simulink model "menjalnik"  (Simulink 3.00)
settings: Solver=ode45  StartTime=0.0  StopTime=100.0  RelTol=1e-3

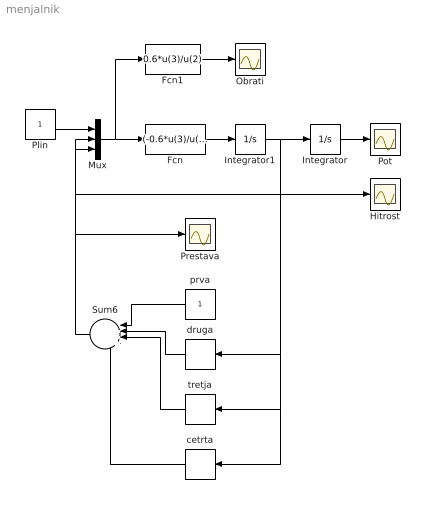
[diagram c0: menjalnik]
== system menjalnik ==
  Fcn : Fcn  Expr=(-0.6*u(3)/u(2)+u(1))/(1+u(2))
  Fcn1 : Fcn  Expr=0.6*u(3)/u(2)
  Hitrost : Scope
  Integrator : Integrator  ExternalReset=none  InitialConditionSource=internal  InitialCondition=0  LimitOutput=off  UpperSaturationLimit=inf  LowerSaturationLimit=-inf  ShowSaturationPort=off  ShowStatePort=off  AbsoluteTolerance=auto
  Integrator1 : Integrator  ExternalReset=none  InitialConditionSource=internal  InitialCondition=0.1  LimitOutput=off  UpperSaturationLimit=inf  LowerSaturationLimit=-inf  ShowSaturationPort=off  ShowStatePort=off  AbsoluteTolerance=auto
  Mux : Mux  Inputs=3
  Obrati : Scope
  Plin : Constant  Value=1
  Pot : Scope
  Prestava : Scope
  Sum6 : Sum  Orientation=left  Inputs=|++++  SaturateOnIntegerOverflow=on
  cetrta : Relay  Orientation=left  OnSwitchValue=4.5  OffSwitchValue=4  OnOutputValue=1  OffOutputValue=0
  druga : Relay  Orientation=left  OnSwitchValue=1.6  OffSwitchValue=1.5  OnOutputValue=1  OffOutputValue=0
  prva : Constant  Orientation=left  Value=1
  tretja : Relay  Orientation=left  OnSwitchValue=3.1  OffSwitchValue=2.9  OnOutputValue=1  OffOutputValue=0
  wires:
  Integrator1/1 -> Integrator/1, druga/1, tretja/1, cetrta/1, Hitrost/1, Mux/3
  Fcn/1 -> Integrator1/1
  Integrator/1 -> Pot/1
  druga/1 -> Sum6/2
  Sum6/1 -> Prestava/1, Mux/2
  Mux/1 -> Fcn/1, Fcn1/1
  prva/1 -> Sum6/1
  Fcn1/1 -> Obrati/1
  Plin/1 -> Mux/1
  tretja/1 -> Sum6/3
  cetrta/1 -> Sum6/4
